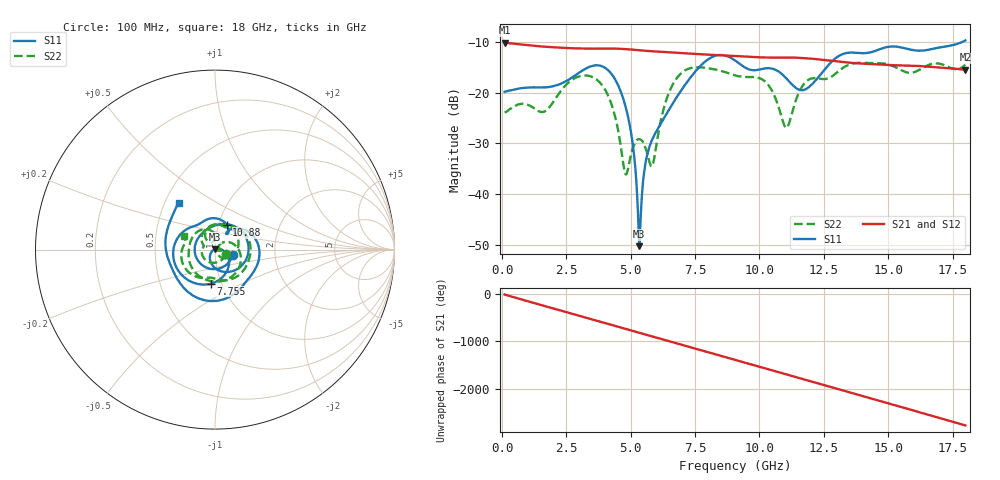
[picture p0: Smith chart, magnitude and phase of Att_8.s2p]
#  HZ  S  DB  R  50.00
! Rohde & Schwarz Vector Network Analyzer
! Rohde-Schwarz,ZNB40-4Port,1311601084101679,3.45
! Created: UTC 4/25/2025, 8:45:12 AM
! freq[Hz]  db:S11  ang:S11  db:S21  ang:S21  db:S12  ang:S12  db:S22  ang:S22
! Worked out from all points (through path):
!   1750 points, 100 MHz to 18 GHz, reference 50 ohm
!   highest |S21| = -10.09 dB at 100 MHz (marker M1); lowest = -15.4 dB at 18 GHz (marker M2)
!   group delay of S21, straight-line fit = 427 ps
!   lowest |S11| = -50.3 dB at 5.33 GHz (marker M3), VSWR 1.01, Z = 49.8 + j0.25 ohm
!   |S11| at or under -10 dB: start of sweep to 17.84 GHz
!   |S22| runs from -36.1 to -14.0 dB; largest |S21 - S12| = 0.00039
!   S11 on the Smith chart (normalised r, x): 100 MHz: 1.21, -0.08; 7.755 GHz: 0.89, -0.35; 10.88 GHz: 1.09, +0.31; 18 GHz: 0.59, +0.34
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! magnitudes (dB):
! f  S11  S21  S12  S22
! 100 MHz  -19.8  -10.1  -10.1  -23.9
! 1.666 GHz  -18.9  -10.9  -10.9  -23.6
! 3.088 GHz  -15.7  -11.2  -11.2  -16.6
! 4.02 GHz  -15.1  -11.2  -11.2  -19.5
! 4.603 GHz  -19.6  -11.3  -11.3  -30.2
! 4.808 GHz  -22.9  -11.3  -11.3  -36.1
! 5.043 GHz  -28.9  -11.4  -11.4  -31.5
! 5.33 GHz  -50.3  -11.6  -11.6  -29.1
! 5.555 GHz  -34.4  -11.7  -11.7  -30.6
! 5.811 GHz  -29.5  -11.8  -11.8  -34.6
! 6.067 GHz  -26.9  -11.8  -11.8  -28.1
! 6.722 GHz  -21.3  -12.0  -12.0  -17.6
! 7.755 GHz  -14.4  -12.4  -12.4  -15.0
! 9.055 GHz  -13.6  -12.7  -12.7  -16.5
! 10.23 GHz  -15.1  -13.0  -13.0  -17.8
! 10.88 GHz  -16.3  -13.0  -13.0  -25.1
! 11.09 GHz  -17.4  -13.0  -13.0  -26.7
! 11.59 GHz  -19.4  -13.1  -13.1  -19.3
! 12.04 GHz  -18.3  -13.2  -13.2  -17.1
! 13.16 GHz  -12.5  -13.8  -13.8  -15.4
! 15.02 GHz  -10.9  -14.5  -14.5  -14.4
! 18 GHz  -9.6  -15.4  -15.4  -14.5
